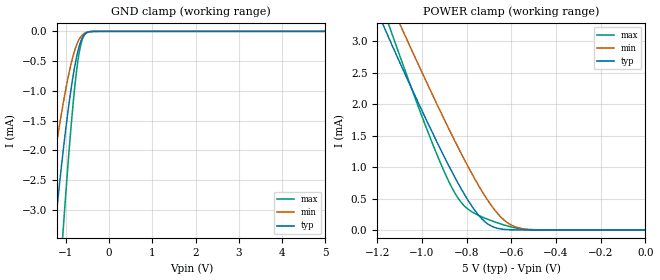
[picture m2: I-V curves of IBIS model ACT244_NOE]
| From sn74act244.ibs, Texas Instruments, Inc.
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[Model]   ACT244_NOE
Model_type  Input
Vinl = 0.8
Vinh = 2
| variable   typ   min   max
C_comp   0.82pF   0.75pF   1.01pF
[Temperature Range]   40   100   -40
| Ambient temperature   25   85   -40
[Voltage range]   5   4.5   5.5
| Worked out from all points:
|   GND clamp passes 1 mA (typ) near -0.89 V on its own axis
|   POWER clamp passes 1 mA (typ) near -0.88 V on its own axis
[GND Clamp]
| ACT244_NOE
|   Voltage   I(typ)   I(min)   I(max)
-5V       -44.02mA   -28.92mA   -56.3mA
-1.5V     -5.247mA   -3.34mA    -8.323mA
-1.295V   -3.627mA   -2.278mA   -5.896mA
-1.245V   -3.258mA   -2.035mA   -5.326mA
-1.07V    -2.061mA   -1.247mA   -3.424mA
-1.05V    -1.934mA   -1.165mA   -3.217mA
-875mV    -948.9uA   -532.8uA   -1.563mA
-765mV    -477.3uA   -254.5uA   -742.5uA
-665mV    -189.7uA   -102uA     -257.4uA
-615mV    -102.4uA   -58.02uA   -125.2uA
-545mV    -35.74uA   -22.48uA   -36.4uA
5V        16.38nA    4.859uA    150.6nA
[POWER Clamp]
| ACT244_NOE
|   Voltage   I(typ)   I(min)   I(max)
-5V       42.78mA    42.05mA    45.9mA
-1.18V    3.317mA    3.918mA    3.588mA
-1.145V   3.031mA    3.64mA     3.233mA
-1.095V   2.633mA    3.247mA    2.732mA
-1.05V    2.283mA    2.896mA    2.289mA
-935mV    1.417mA    2.018mA    1.219mA
-840mV    755.6uA    1.327mA    515.7uA
-795mV    479.5uA    1.018mA    334uA
-730mV    170uA      608.8uA    206.3uA
-625mV    7.61uA     135.7uA    71.71uA
-505mV    124.6nA    5.639uA    1.54uA
-84.45fV  16.38nA    947.5pA    229.7nA
